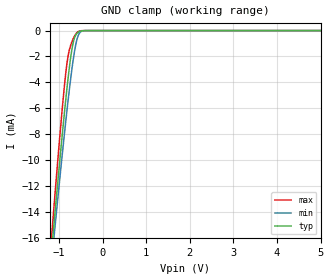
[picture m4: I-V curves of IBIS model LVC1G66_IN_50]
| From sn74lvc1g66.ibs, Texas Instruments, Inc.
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[Model]   LVC1G66_IN_50
Model_type  Input
Vinl=1.35
Vinh=3.85
| variable   typ   min   max
C_comp   2.82pF   2.47pF   3.31pF
[Temperature Range]   40   100   -40
| Ambient temperature   25   85   -40
[Voltage range]   5   4.5   5.5
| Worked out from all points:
|   GND clamp passes 1 mA (typ) near -0.68 V on its own axis
[GND Clamp]
| LVC1G66_IN_50
|   Voltage   I(typ)   I(min)   I(max)
-5.5V     -200.6mA   -187.3mA   -217mA
-1.16V    -16.65mA   -17.52mA   -15.49mA
-1.125V   -15.33mA   -16.31mA   -14.02mA
-1.09V    -14.01mA   -15.1mA    -12.56mA
-925mV    -8.038mA   -9.561mA   -6.02mA
-815mV    -4.394mA   -6.099mA   -2.476mA
-765mV    -2.925mA   -4.629mA   -1.532mA
-685mV    -1.105mA   -2.511mA   -711.6uA
-610mV    -316.3uA   -993uA     -240.8uA
-545mV    -93.69uA   -277.9uA   -57.03uA
-280mV    -74.48nA   -223.6nA   -3.9nA
5V        94.34pA    195.1pA    60.23pA
